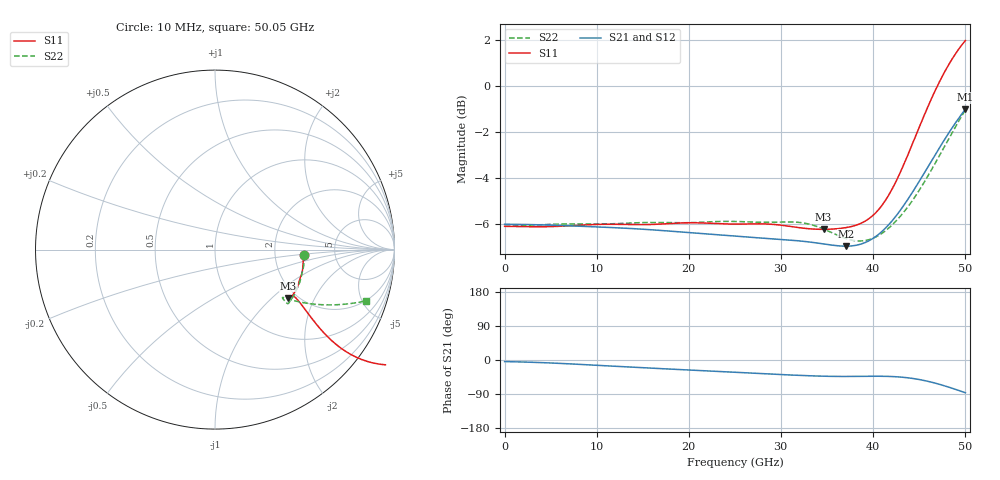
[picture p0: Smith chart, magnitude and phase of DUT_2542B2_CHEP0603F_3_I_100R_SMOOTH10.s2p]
! Touchstone file from project
! Exported from ElectronicsDesktop 2025.1.3
# GHz S MA R 50.000000
! Terminal data exported
! Port[1] = Port1
! Port[2] = Port2
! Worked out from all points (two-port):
!   144 points, 10 MHz to 50.05 GHz, reference 50 ohm
!   highest |S21| = -1.01 dB at 50.05 GHz (marker M1); lowest = -6.9 dB at 37.1 GHz (marker M2)
!   |S21| within 3 dB of the highest: 45.23 GHz to end of sweep
!   lowest |S11| = -6.2 dB at 34.66 GHz (marker M3), VSWR 2.91, Z = 90 - j63.7 ohm
!   |S11| at or under -10 dB: nowhere
!   |S22| runs from -6.7 to -1.0 dB; largest |S21 - S12| = 0.0038
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0.01  0.4964 -3.4  0.5016 -4.2  0.5008 -3.9  0.4963 -3.6
! Gamma 0 0 0 0
! Port Impedance 50 0 50 0
4.2094  0.4955 -6.7  0.5 -7.0  0.4986 -6.9  0.5007 -6.9
8.4088  0.4995 -11.7  0.4965 -11.8  0.4949 -11.8  0.5022 -12.1
16.8076  0.5019 -21.7  0.4866 -22.6  0.4858 -22.6  0.506 -22.9
21.35695  0.5049 -26.2  0.4789 -28.0  0.4787 -28.0  0.5066 -28.0
25.2064  0.502 -29.6  0.4726 -32.7  0.4725 -32.7  0.5086 -31.2
30.8056  0.4969 -32.5  0.4638 -39.3  0.4638 -39.3  0.5076 -36.0
33.6052  0.4896 -33.5  0.4578 -42.0  0.4576 -42.1  0.4985 -36.7
34.65505  0.489 -33.4  0.4547 -42.8  0.4544 -42.8  0.4898 -36.5
37.1047  0.4933 -31.9  0.4497 -43.5  0.4492 -43.5  0.467 -35.9
38.85445  0.5055 -30.8  0.4554 -43.1  0.4549 -43.2  0.4617 -35.3
39.9043  0.5218 -30.8  0.4659 -42.9  0.4654 -42.9  0.4668 -34.9
40.95415  0.5498 -31.7  0.4832 -42.9  0.4826 -42.9  0.4788 -34.4
42.004  0.5932 -33.3  0.5078 -43.6  0.5072 -43.5  0.4978 -33.8
43.05385  0.6543 -35.2  0.5401 -45.1  0.5393 -45.1  0.5238 -32.9
44.1037  0.7324 -36.9  0.5799 -47.9  0.579 -47.8  0.5573 -31.6
45.5035  0.8561 -38.1  0.6435 -53.7  0.6424 -53.6  0.6148 -29.4
46.55335  0.9557 -37.7  0.6974 -59.7  0.6961 -59.5  0.6678 -27.4
47.6032  1.054 -36.3  0.7547 -66.8  0.7532 -66.6  0.7282 -25.0
48.3031  1.116 -34.9  0.7937 -72.1  0.7921 -71.9  0.7718 -23.3
49.003  1.175 -33.2  0.8327 -77.7  0.831 -77.5  0.8172 -21.5
50.05285  1.254 -30.4  0.8901 -86.5  0.8882 -86.2  0.8873 -18.8
